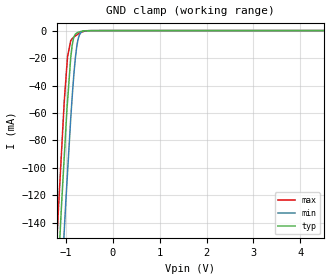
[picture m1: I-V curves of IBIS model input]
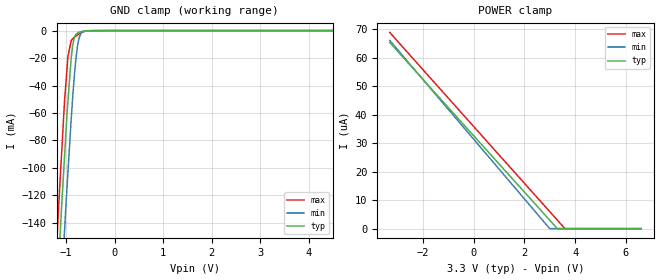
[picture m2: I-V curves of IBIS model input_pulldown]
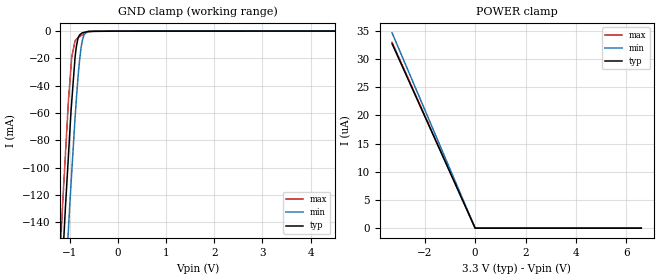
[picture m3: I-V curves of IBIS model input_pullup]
|Texas Instruments Incorporated
| Integrated Analog Front End for Pulse Oximeters
| Marketing part#   Digital Voltage Range   Package-type   #pins
| AFE4490RHAR   2.0V -3.6V   VQFN   40
| AFE4490RHAT   2.0V -3.6V   VQFN   40
[IBIS Ver]   4.1
[File name]   afe4490.ibs
[File Rev]   1.0
[Date]   2/12/2013
[Source]
| Texas Instruments Incorporated.
| Analog-eLab Design Center, HPA
| 12500 TI Blvd
| Dallas, TX -75243
[Notes]   Revision History:
| Rev 1.0: 2/12/2013
| - Initial version of the model
| - Model generated from simulations in TISPICE
| - Model matched to SPICE simulation
| - C_comp although listed in numerical order of value are
|   obtained from varying PVT conditions. For PVT conditions for
|   each specific value refer the buffer description under
|   respective [Model]. IBIS model user is responsible for using
|   appropriate C_comp to simulate for Signal Integrity.
|*   EXCEPTION:   *
|*   - For model input_pulldown,there will be small leakage current in POWER *
|*   Clamp IV table because of a pulldown resistor R0  connected to PAD.  *
|*   - For model input_pullup,there will be  small leakage current in GND   *
|*   Clamp IV table because of a pullup resistor R0  connected to PAD.   *
[Disclaimer]
| This model is designed as an aid for customers of Texas Instruments.
| TI and its licensors and suppliers make no warranties, either expressed
| or implied, with respect to this  model, including the warranties of
| merchantability or fitness for a particular purpose. The model is
| provided solely on an "as is" basis. The entire risk as to its quality
| and performance is with the customer.
[Copyright]
(C) Copyright 2013 Texas Instruments Incorporated.All rights reserved.
|   AFE4490RHA
[Component]   AFE4490RHA
[Manufacturer]   TI
[Package]   |40 VQFN  -  RHA package
|   typ   min   max
R_pkg   0.134095   0.11611   0.16206
L_pkg   1.737375nH   1.48032nH   2.13924nH
C_pkg   0.130051pF   0.11707pF   0.15079pF
[Pin]  signal_name   model_name   R_pin   L_pin   C_pin
1   INN   nc   0.14238   1.86243nH  0.13319pF
2   INP   nc   0.12719   1.64475nH  0.12665pF
3   RX_ANA_GND   gnd   0.11986   1.54066nH  0.11470pF
4   VCM   nc   0.13784   1.79602nH  0.13117pF
5   DNC   nc   0.12417   1.60161nH  0.12500pF
6   DNC   nc   0.11755   1.50812nH  0.11929pF
7   BG   nc   0.11727   1.50413nH  0.12015pF
8   VSS   gnd   0.12488   1.61177nH  0.12500pF
9   TX_REF   nc   0.13518   1.75836nH  0.13180pF
10   DNC   nc   0.14839   1.94844nH  0.13452pF
11   TX_CTRL_SUP   power   0.15360   2.02333nH  0.13364pF
12   LED_DRV_GND   gnd   0.09225   1.98726nH  0.23355pF
13   LED_DRV_GND   gnd   0.08390   1.75667nH  0.23411pF
14   TXN   nc   0.07917   1.62443nH  0.21992pF
15   TXP   nc   0.07266   1.44918nH  0.20589pF
16   LED_DRV_GND   gnd   0.12038   1.54582nH  0.12580pF
17   LED_DRV_SUP   power   0.07057   1.39691nH  0.19623pF
18   LED_DRV_SUP   power   0.07170   1.39831nH  0.19503pF
19   RX_DIG_GND   gnd   0.12147   1.55886nH  0.11923pF
20   AFE_PDN   input   0.14414   1.88264nH  0.13407pF
21   DIAD_END   outp   0.15046   1.97233nH  0.14028pF
22   LED_ALM   outp   0.13741   1.78385nH  0.13394pF
23   PD_ALM/ADC_Reset outp   0.12607   1.62186nH  0.12182pF
24   SCLK   input_pulldown   0.12571   1.61662nH  0.12048pF
25   SPISOMI   outp   0.11859   1.51551nH  0.11815pF
26   SPISIMO   input_pulldown   0.11611   1.48032nH  0.11707pF
27   SPISTE   input_pullup   0.12024   1.53893nH  0.12061pF
28   ADC_RDY   outp   0.12978   1.67477nH  0.12967pF
29   _RESET   input_pullup   0.14448   1.88506nH  0.14369pF
30   CLKOUT   outp   0.16206   2.13924nH  0.15079pF
31   RX_DIG_GND   gnd   0.07163   1.49683nH  0.17036pF
32   RX_DIG_GND   gnd   0.06117   1.18479nH  0.16759pF
33   RX_ANA_SUP   power   0.05850   1.10874nH  0.15946pF
34   RXOUTN   nc   0.11614   1.48482nH  0.11820pF
35   RXOUTP   nc   0.12179   1.56581nH  0.12459pF
36   RX_ANA_GND   gnd   0.13508   1.75582nH  0.13216pF
37   XOUT   nc   0.13940   1.81783nH  0.12934pF
38   XIN   nc   0.14033   1.83107nH  0.12907pF
39   RX_ANA_SUP   power   0.06706   1.33079nH  0.17101pF
40   RX_ANA_GND   gnd   0.14917   1.95954nH  0.14164pF
| Models and submodels in the file (4): input (Input), input_pulldown (Input), input_pullup (Input), outp (Output)
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|   input Model
[Model]   input
Model_type   Input
Vinl = 0.6
Vinh = 2.4
|   typ   min   max
|   (nom PVT)   (fast PVT)   (slow PVT)
C_comp   3.312e-13   3.289e-13   3.358e-13
[Model spec]
|subparameter
Vinl   0.66   0.6   0.72
Vinh   2.64   2.4   2.88
| Where nom  PVT is Nominal Process, 3.3V, 27C
|   Fast PVT is Strong Process,  3.6V, -40C
|   Slow PVT is Weak Process,   3V, 105C
[Voltage Range]   3.3   3   3.6
|Junction Temperature
[Temperature Range]   27   105   -40
[Power Clamp Reference]   3.3   3   3.6
[GND Clamp Reference]   0   0   0
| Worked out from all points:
|   GND clamp passes 1 mA (typ) near -0.72 V on its own axis
[GND Clamp]
|   Voltage   I(typ)   I(min)   I(max)
-3.3V     -1.734A    -1.762A    -1.725A
-1.27V    -245.7mA   -302.2mA   -207.4mA
-1.156V   -168.6mA   -223.4mA   -127.4mA
-1.137V   -156.2mA   -210.7mA   -115.7mA
-1.099V   -130.6mA   -186.4mA   -91.68mA
-1.037V   -92.87mA   -146.8mA   -52.56mA
-964.8mV  -51.35mA   -103.1mA   -18.88mA
-897.6mV  -19.84mA   -64.25mA   -7.375mA
-825mV    -4.345mA   -29.78mA   -4.502mA
-745.8mV  -1.232mA   -7.144mA   -2.676mA
-591mV    -190.8uA   -137.2uA   -416.9uA
6.6V      0A         0A         0A
[POWER Clamp]
|   Voltage   I(typ)   I(min)   I(max)
-3.3V     0A         0A         0A
0V        0A         0A         0A
6.6V      0A         0A         0A
|   input_pulldown Model
[Model]   input_pulldown
Model_type   Input
Vinl = 0.6
Vinh = 2.4
|   typ   min   max
|   (nom PVT)   (fast PVT)   (slow PVT)
C_comp   3.312e-13   3.289e-13   3.358e-13
[Model spec]
|subparameter
Vinl   0.66   0.6   0.72
Vinh   2.64   2.4   2.88
| Where nom  PVT is Nominal Process, 3.3V, 27C
|   Fast PVT is Strong Process,  3.6V, -40C
|   Slow PVT is Weak Process,   3V, 105C
[Voltage Range]   3.3   3   3.6
|Junction Temperature
[Temperature Range]   27   105   -40
[Power Clamp Reference]   3.3   3   3.6
[GND Clamp Reference]   0   0   0
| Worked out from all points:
|   GND clamp passes 1 mA (typ) near -0.72 V on its own axis
[GND Clamp]
|   Voltage   I(typ)   I(min)   I(max)
-3.3V     -1.734A    -1.762A    -1.725A
-1.27V    -245.7mA   -302.2mA   -207.4mA
-1.156V   -168.6mA   -223.4mA   -127.4mA
-1.137V   -156.2mA   -210.7mA   -115.7mA
-1.099V   -130.6mA   -186.4mA   -91.68mA
-1.037V   -92.87mA   -146.8mA   -52.57mA
-964.8mV  -51.35mA   -103.1mA   -18.88mA
-897.6mV  -19.84mA   -64.26mA   -7.379mA
-825mV    -4.348mA   -29.78mA   -4.505mA
-745.8mV  -1.237mA   -7.146mA   -2.68mA
-591mV    -195.8uA   -141.5uA   -421.6uA
6.6V      0A         0A         0A
[POWER Clamp]
|   Voltage   I(typ)   I(min)   I(max)
-3.3V     65.41uA    66.12uA    68.93uA
2.997V    3uA        31.46nA    6.017uA
3.297V    32.67nA    0A         3.027uA
3.604V    0A         0A         0A
6.6V      0A         0A         0A
|   input_pullup Model
[Model]   input_pullup
Model_type   Input
Vinl = 0.6
Vinh = 2.4
|   typ   min   max
|   (nom PVT)   (fast PVT)   (slow PVT)
C_comp   3.312e-13   3.289e-13   3.358e-13
[Model spec]
|subparameter
Vinl   0.66   0.6   0.72
Vinh   2.64   2.4   2.88
| Where nom  PVT is Nominal Process, 3.3V, 27C
|   Fast PVT is Strong Process,  3.6V, -40C
|   Slow PVT is Weak Process,   3V, 105C
[Voltage Range]   3.3   3   3.6
|Junction Temperature
[Temperature Range]   27   105   -40
[Power Clamp Reference]   3.3   3   3.6
[GND Clamp Reference]   0   0   0
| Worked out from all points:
|   GND clamp passes 1 mA (typ) near -0.71 V on its own axis
[GND Clamp]
|   Voltage   I(typ)   I(min)   I(max)
-3.3V     -1.734A    -1.762A    -1.725A
-1.27V    -245.7mA   -302.2mA   -207.4mA
-1.156V   -168.6mA   -223.4mA   -127.4mA
-1.137V   -156.2mA   -210.7mA   -115.7mA
-1.099V   -130.6mA   -186.4mA   -91.69mA
-1.037V   -92.88mA   -146.8mA   -52.58mA
-964.8mV  -51.36mA   -103.1mA   -18.9mA
-881.1mV  -14.53mA   -55.87mA   -6.602mA
-798mV    -2.701mA   -19.89mA   -3.904mA
-745.8mV  -1.258mA   -7.155mA   -2.702mA
-591mV    -235.2uA   -166.6uA   -451.7uA
6.6V      0A         0A         0A
[POWER Clamp]
|   Voltage   I(typ)   I(min)   I(max)
-3.3V     32.68uA    34.62uA    32.94uA
-1.911V   18.92uA    20.04uA    19.07uA
-33.83fV  0A         0A         0A
6.6V      0A         0A         0A
